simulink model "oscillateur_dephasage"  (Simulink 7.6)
settings: Solver=ode15s  StartTime=0.0  StopTime=30  RelTol=1e-3
InitFcn:
  | clc, close all
  | C=0.01e-3;
  | R=1e3;
StopFcn:
  | close all, clc
  | load oscillateur.mat
  | plot(x(1,:),x(2,:))
  | title('Oscillateur à déphasage')
  | xlabel('temps')
  | grid
libraries: fl_lib x10, nesl_utility x3, elec_lib x1

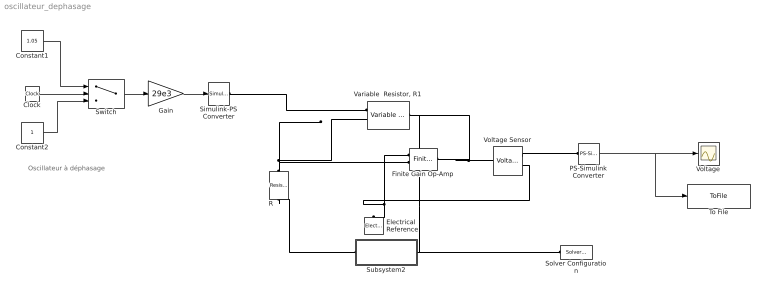
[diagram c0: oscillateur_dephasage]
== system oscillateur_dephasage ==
  note: Oscillateur à déphasage
  Clock : Clock
  Constant1 : Constant  Value=1.05
  Constant2 : Constant
  Electrical Reference : fl_lib/Electrical/Electrical Elements/Electrical Reference  DialogController=NetworkEngine.DynNeDlgSource  SystemSampleTime=-1  i_Log=off  LocalVarNames=|i  LocalVarDescs=|i  LocalVarLogging=[]
  Finite Gain Op-Amp : elec_lib/Integrated Circuits/Finite Gain Op-Amp  DialogController=NetworkEngine.DynNeDlgSource  SystemSampleTime=-1  A=1000  Rin=1e+06 Ohm  Rout=100 Ohm  Vmin=-15 V  Vmax=15 V  LocalVarNames=|power  LocalVarDescs=|Dissipated power (W)  LocalVarLogging=0
  Gain : Gain  Gain=29e3
  PS-Simulink Converter : nesl_utility/PS-Simulink Converter  DialogController=NetworkEngine.DynNeUtilDlgSource  SystemSampleTime=-1  PhysicalDomain=network_engine_domain  LeftPortType=input  RightPortType=output  SubClassName=ps_output  Unit=1  AffineConversion=off
  R : fl_lib/Electrical/Electrical Elements/Resistor  DialogController=NetworkEngine.DynNeDlgSource  SystemSampleTime=-1  R=1 kOhm  i_Log=off  v_Log=off  LocalVarNames=|current|voltage|power  LocalVarDescs=|Resistor current (A)|Voltage across resistor (V)|Power (W)  LocalVarLogging=[0 0 0]
  Simulink-PS Converter : nesl_utility/Simulink-PS Converter  DialogController=NetworkEngine.DynNeUtilDlgSource  SystemSampleTime=-1  PhysicalDomain=network_engine_domain  LeftPortType=input  RightPortType=output  SubClassName=ps_input  Unit=1  AffineConversion=off  InputFilterTimeConstant=.001  UdotUserProvided=0
  Solver Configuration : nesl_utility/Solver Configuration  DialogController=NetworkEngine.DynNeUtilDlgSource  SystemSampleTime=-1  PhysicalDomain=network_engine_domain  LeftPortType=input  RightPortType=generic  SubClassName=solver  Accelerate=off  Profile=off  ResidualTolerance=1e-9  MaxNonlinIter=12  MaxModeIter=2  DoFixedCost=off  UseLocalSampling=off  DoDC=off  LinearAlgebra=Sparse  LocalSolverSampleTime=.001  LocalSolverChoice=NE_BACKWARD_EULER_ADVANCER  UseLocalSolver=off
  Subsystem2 : Subsystem
  Switch : Switch  Threshold=25
  To File : ToFile  Filename=oscillateur.mat  MatrixName=x
  "Variable  Resistor, R1" : fl_lib/Electrical/Electrical Elements/Variable Resistor  DialogController=NetworkEngine.DynNeDlgSource  SystemSampleTime=-1  Rmin=0 Ohm  i_Log=off  v_Log=off  LocalVarNames=|i|v  LocalVarDescs=|i|v  LocalVarLogging=[0 0]
  Voltage : Scope
  Voltage Sensor : fl_lib/Electrical/Electrical Sensors/Voltage Sensor  DialogController=NetworkEngine.DynNeDlgSource  SystemSampleTime=-1  i1_Log=off  v1_Log=off  LocalVarNames=|i1|v1  LocalVarDescs=|i1|v1  LocalVarLogging=[]
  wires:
  PS-Simulink Converter/1 -> Voltage/1, To File/1
  Gain/1 -> Simulink-PS Converter/1
  Switch/1 -> Gain/1
  Clock/1 -> Switch/2
  Constant1/1 -> Switch/1
  Constant2/1 -> Switch/3
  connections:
  "Variable  Resistor, R1"/RConn1 -- Finite Gain Op-Amp/RConn1 -- Voltage Sensor/LConn1 -- Subsystem2/LConn1 -- Solver Configuration/RConn1
  Voltage Sensor/RConn1 -- PS-Simulink Converter/LConn1
  R/LConn1 -- Finite Gain Op-Amp/LConn2 -- "Variable  Resistor, R1"/LConn2
  Finite Gain Op-Amp/LConn1 -- Electrical Reference/LConn1 -- Voltage Sensor/RConn2
  Subsystem2/RConn1 -- R/RConn1
  Simulink-PS Converter/RConn1 -- "Variable  Resistor, R1"/LConn1

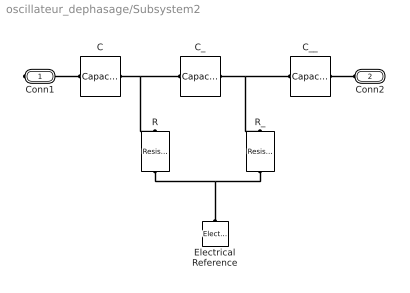
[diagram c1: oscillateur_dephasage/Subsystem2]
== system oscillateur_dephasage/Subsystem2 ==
  C : fl_lib/Electrical/Electrical Elements/Capacitor  DialogController=NetworkEngine.DynNeDlgSource  SystemSampleTime=-1  c=C F  v0=0.5 V  r=0 Ohm  g=0 1/Ohm  i_Log=off  v_Log=off  vc_Log=off  LocalVarNames=|i|v|vc  LocalVarDescs=|i|v|Internal variable for voltage across capacitor term  LocalVarLogging=[0 0 0]
  C_ : fl_lib/Electrical/Electrical Elements/Capacitor  DialogController=NetworkEngine.DynNeDlgSource  SystemSampleTime=-1  c=C F  v0=0 V  r=0 Ohm  g=0 1/Ohm  i_Log=off  v_Log=off  vc_Log=off  LocalVarNames=|i|v|vc  LocalVarDescs=|i|v|Internal variable for voltage across capacitor term  LocalVarLogging=[0 0 0]
  C__ : fl_lib/Electrical/Electrical Elements/Capacitor  DialogController=NetworkEngine.DynNeDlgSource  SystemSampleTime=-1  c=C F  v0=0 V  r=0 Ohm  g=0 1/Ohm  i_Log=off  v_Log=off  vc_Log=off  LocalVarNames=|i|v|vc  LocalVarDescs=|i|v|Internal variable for voltage across capacitor term  LocalVarLogging=[0 0 0]
  Electrical Reference : fl_lib/Electrical/Electrical Elements/Electrical Reference  DialogController=NetworkEngine.DynNeDlgSource  SystemSampleTime=-1  i_Log=off  LocalVarNames=|i  LocalVarDescs=|i  LocalVarLogging=[]
  R : fl_lib/Electrical/Electrical Elements/Resistor  DialogController=NetworkEngine.DynNeDlgSource  SystemSampleTime=-1  R=R Ohm  i_Log=off  v_Log=off  LocalVarNames=|current|voltage|power  LocalVarDescs=|Resistor current (A)|Voltage across resistor (V)|Power (W)  LocalVarLogging=[0 0 0]
  R_ : fl_lib/Electrical/Electrical Elements/Resistor  DialogController=NetworkEngine.DynNeDlgSource  SystemSampleTime=-1  R=R Ohm  i_Log=off  v_Log=off  LocalVarNames=|current|voltage|power  LocalVarDescs=|Resistor current (A)|Voltage across resistor (V)|Power (W)  LocalVarLogging=[0 0 0]
  Conn1 : PMIOPort  Port=1  Side=Right
  Conn2 : PMIOPort  Port=2  Side=Left
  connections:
  C/LConn1 -- C_/RConn1 -- R/LConn1
  C_/LConn1 -- C__/RConn1 -- R_/LConn1
  R/RConn1 -- Electrical Reference/LConn1 -- R_/RConn1
  Conn1/RConn1 -- C/RConn1
  Conn2/RConn1 -- C__/LConn1
